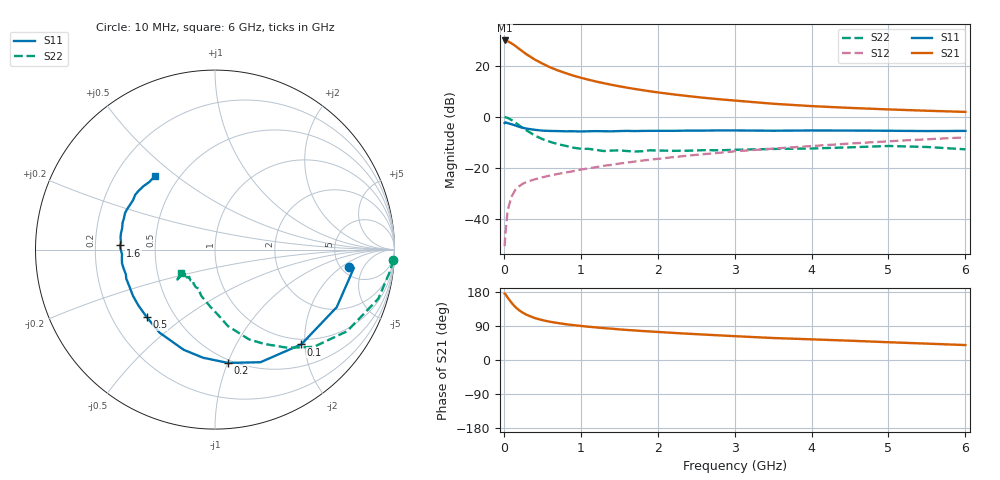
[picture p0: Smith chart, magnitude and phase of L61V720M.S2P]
!  INFINEON TECHNOLOGIES Small Signal Semiconductors
! BFR380L3 , Si-NPN RF-Transistor in TSLP-3-1
!  Vce=1.75 V,  Ic=20 mA
! Common Emitter S-Parameters:  07. March 2005
#  GHz  S  MA  R  50
! f  S11  S21  S12  S22
! GHz  Mag  Ang  Mag  Ang  Mag  Ang  Mag  Ang
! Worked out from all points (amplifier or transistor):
!   36 points, 10 MHz to 6 GHz, reference 50 ohm
!   highest |S21| = 30.0 dB at 10 MHz (marker M1)
!   |S21| within 3 dB of that: start of sweep to 186.3 MHz
!   unconditionally stable (mu >= 1): 1.927 GHz to 4.882 GHz
!   at 250 MHz: K = 0.35, MSG = 25.9 dB, |S12| = -26.2 dB
!   at 1.4 GHz: K = 0.95, MSG = 15.7 dB, |S12| = -18.9 dB
!   at 6 GHz: K = 0.98, MSG = 5.0 dB, |S12| = -8.1 dB
!   S11 on the Smith chart (normalised r, x): 10 MHz: 5.91, -2.72; 100 MHz: 0.89, -1.93; 200 MHz: 0.47, -1.00; 500 MHz: 0.35, -0.37; 1.6 GHz: 0.31, +0.02; 6 GHz: 0.37, +0.42
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0.01  0.7558 -7.5  31.45 175.0  0.0029 83.4  0.9957 -3.3
0.02  0.7803 -7.6  31.2 174.0  0.0051 82.0  0.983 -7.0
0.05  0.7503 -25.3  30.34 164.5  0.0147 80.0  0.9504 -16.7
0.1  0.7141 -47.7  27.64 151.1  0.0272 69.6  0.8654 -31.7
0.15  0.6768 -68.0  24.53 139.7  0.0372 61.4  0.7722 -44.6
0.2  0.6354 -83.5  21.46 131.0  0.0437 57.0  0.6794 -53.6
0.25  0.6061 -96.3  18.88 124.4  0.0489 53.1  0.5931 -62.4
0.3  0.5849 -107.3  16.62 118.9  0.0532 51.2  0.5354 -69.2
0.4  0.5565 -123.8  13.37 110.8  0.0592 49.3  0.4321 -80.4
0.5  0.5351 -135.2  11.08 105.3  0.0649 49.5  0.3657 -87.1
0.6  0.5282 -143.9  9.372 100.9  0.0705 50.2  0.3238 -93.9
0.8  0.5193 -156.7  7.21 94.6  0.0808 52.9  0.2701 -106.2
0.9  0.5203 -161.8  6.434 92.1  0.0856 54.3  0.248 -110.7
1.1  0.52 -168.4  5.339 87.8  0.0978 56.3  0.2353 -117.0
1.3  0.5209 -175.1  4.564 84.1  0.1095 57.6  0.2129 -124.6
1.6  0.5294 177.5  3.732 79.3  0.1263 59.2  0.2132 -132.6
2.2  0.5308 167.0  2.758 71.6  0.1616 61.2  0.2153 -136.4
2.8  0.5408 157.9  2.211 65.0  0.1969 62.1  0.2203 -142.8
3.5  0.5333 149.0  1.804 58.0  0.2371 60.8  0.2343 -142.3
4.5  0.537 142.5  1.495 50.9  0.2989 59.7  0.252 -142.1
5.5  0.5253 134.2  1.315 43.2  0.3624 56.4  0.2557 -142.3
6  0.5291 128.9  1.248 39.4  0.3949 54.4  0.2303 -145.1
